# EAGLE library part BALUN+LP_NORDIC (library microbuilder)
Balun + Low Pass Filter 0603 Johanson 2450BM14A0002 (nRF8001) - 2400-2500 MHz Balun + Filter
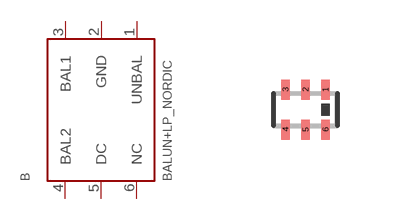
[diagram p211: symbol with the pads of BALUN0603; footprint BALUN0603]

Designator prefix B

## BALUN+LP_NORDIC  [BALUN0603]
1  UNBAL
2  GND  sup
3  BAL1
4  BAL2
5  DC
6  NC  nc

## Footprint BALUN0603 (pad centres in mm)
smd 0.2 x 0.5: 1 0.5,0.5; 2 0,0.5; 3 -0.5,0.5; 4 -0.5,-0.5; 5 0,-0.5; 6 0.5,-0.5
